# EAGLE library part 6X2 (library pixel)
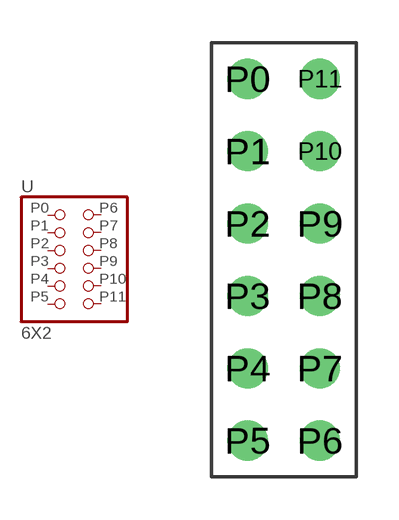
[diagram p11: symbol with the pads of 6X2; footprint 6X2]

Designator prefix -

## 6X2  [6X2]
P0  P0  pas
P1  P1  pas
P2  P2  pas
P3  P3  pas
P4  P4  pas
P5  P5  pas
P6  P6  pas
P7  P7  pas
P8  P8  pas
P9  P9  pas
P10  P10  pas
P11  P11  pas

## Footprint 6X2 (pad centres in mm)
drill 0.9 pad 1.27: P0 -1.27,6.35; P1 -1.27,3.81; P2 -1.27,1.27; P3 -1.27,-1.27; P4 -1.27,-3.81; P5 -1.27,-6.35; P6 1.27,-6.35; P7 1.27,-3.81; P8 1.27,-1.27; P9 1.27,1.27; P10 1.27,3.81; P11 1.27,6.35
